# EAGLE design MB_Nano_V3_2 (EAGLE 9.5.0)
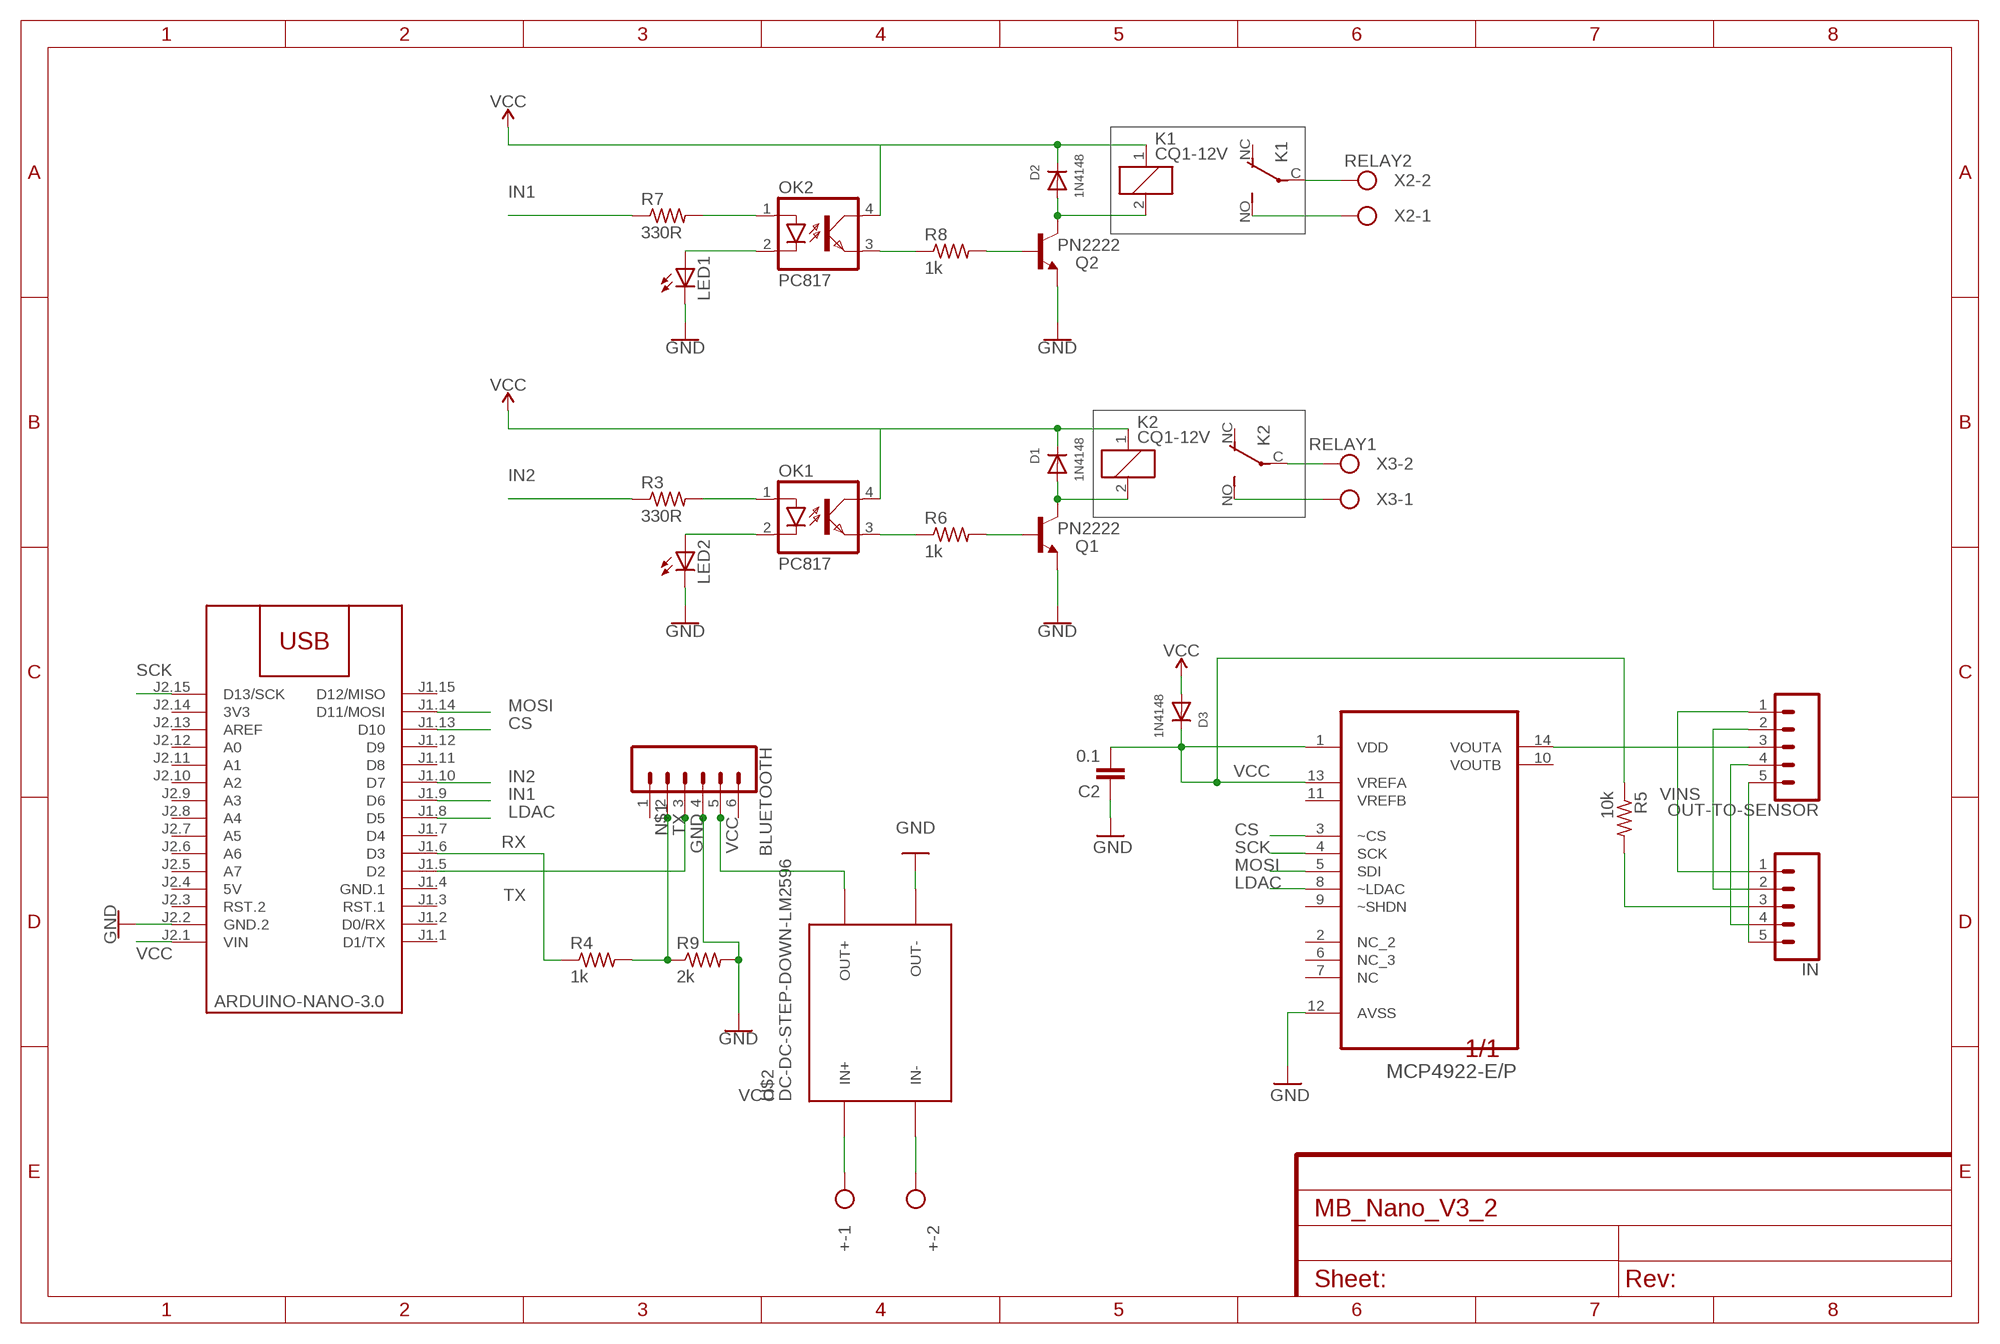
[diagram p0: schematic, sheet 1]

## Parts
+  Vcc  W237-102  [W237-102]
BLUETOOTH  CONN_06LONGPADS  [1X06_LONGPADS]
C2  0.1  CAPPTH1  [CAP-PTH-5MM]
D1  1N4148  DIODEDO-1N4148  [DO-1N4148]
D2  1N4148  DIODEDO-1N4148  [DO-1N4148]
D3  1N4148  DIODEDO-1N4148  [DO-1N4148]
IN  CONN_05PTH_LONGPADS  [1X05_LONGPADS]
K1  CQ1-12V  [CQ1]
K2  CQ1-12V  [CQ1]
LED1  LED3MM  [LED3MM]
LED2  LED3MM  [LED3MM]
M2  ARDUINO-NANO-3.0  [ARDUINO-NANO-3.0]
OK1  PC817  [DIL04]
OK2  PC817  [DIL04]
OUT-TO-SENSOR  CONN_05PTH_LONGPADS  [1X05_LONGPADS]
Q1  PN2222  BC447  [TO92-EBC]
Q2  PN2222  BC447  [TO92-EBC]
R3  330R  R-US_0204/7  [0204/7]
R4  1k  R-US_0204/7  [0204/7]
R5  10k  R-US_0204/7  [0204/7]
R6  1k  R-US_0204/7  [0204/7]
R7  330R  R-US_0204/7  [0204/7]
R8  1k  R-US_0204/7  [0204/7]
R9  2k  R-US_0204/7  [0204/7]
U$2  DC-DC-STEP-DOWN-LM2596  [DC-DC-STEP-DOWN-LM2596]
U$3  MCP4922-E/P  [DIP254P762X533-14]
X2  RELAY2  W237-102  [W237-102]
X3  RELAY1  W237-102  [W237-102]

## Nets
1: IN.5 OUT-TO-SENSOR.5
2: IN.4 OUT-TO-SENSOR.4
4: IN.2 OUT-TO-SENSOR.2
5: IN.1 OUT-TO-SENSOR.1
22: D2.A K1.2 Q2.C
+: +.1 U$2.IN+
-: +.2 U$2.IN-
CS: M2.J1.13(D10) U$3.3(~CS)
GND: BLUETOOTH.4 C2.1 LED1.K(C) LED2.K(C) M2.J2.2(GND.2) Q1.E Q2.E R9.2 U$2.OUT- U$3.12(AVSS)
GND-: D1.A K2.2 Q1.C
IN1: M2.J1.9(D6) R7.1
IN2: M2.J1.10(D7) R3.1
INS: OK1.1(A) R3.2
INSS: OK2.1(A) R7.2
LDAC: M2.J1.8(D5) U$3.8(~LDAC)
LED: LED2.A OK1.2(C)
LEDS: LED1.A OK2.2(C)
MOSI: M2.J1.14(D11/MOSI) U$3.5(SDI)
N$1: BLUETOOTH.2 R4.2 R9.1
N$2: K1.NO(2:S) X2.1
N$3: K1.C(2:P) X2.2
N$4: K2.NO(2:S) X3.1
N$5: K2.C(2:P) X3.2
N$12: Q1.B R6.2
N$20: Q2.B R8.2
N$22: OK2.3(EMIT) R8.1
OTP: OK1.3(EMIT) R6.1
RX: M2.J1.6(D3) R4.1
SCK: M2.J2.15(D13/SCK) U$3.4(SCK)
TX: BLUETOOTH.3 M2.J1.5(D2)
VCC: BLUETOOTH.5 C2.2 D1.C D2.C D3.A D3.C K1.1 K2.1 M2.J2.1(VIN) OK1.4(COL) OK2.4(COL) R5.1 U$2.OUT+ U$3.1(VDD) U$3.13(VREFA)
VINS: IN.3 R5.2
VOUT: OUT-TO-SENSOR.3 U$3.14(VOUTA)
Unconnected: BLUETOOTH.1 BLUETOOTH.6 K1.NC(2:O) K2.NC(2:O) M2.J1.1(D1/TX) M2.J1.2(D0/RX) M2.J1.3(RST.1) M2.J1.7(D4) M2.J1.11(D8) M2.J1.12(D9) M2.J1.15(D12/MISO) M2.J2.3(RST.2) M2.J2.5(A7) M2.J2.6(A6) M2.J2.7(A5) M2.J2.8(A4) M2.J2.9(A3) M2.J2.10(A2) M2.J2.11(A1) M2.J2.12(A0) M2.J2.13(AREF) U$3.2(NC_2) U$3.6(NC_3) U$3.7(NC) U$3.9(~SHDN) U$3.10(VOUTB) U$3.11(VREFB)

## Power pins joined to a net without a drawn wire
3V3: M2.J2.14(3V3)
5V: M2.J2.4(5V)
GND.1: M2.J1.4(GND.1)

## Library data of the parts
+ X2 X3 = con-wago-500:W237-102: WAGO SCREW CLAMP; MPN: 237-102; OC_FARNELL: unknown; OC_NEWARK: 70K9898
BLUETOOTH = SparkFun-Connectors:CONN_06: Multi connection point. Often used as Generic Header-pin footprint for 0.1 inch spaced/style header connections On any of the 0.1 inch spaced packages, you can populate with these: Break Away Headers - Straight (PRT-00116) Break Away Male Headers - Right Angle (PRT-00553) Female Headers (PRT-00115)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
C2 = SparkFun-Passives:CAP: Capacitor
D1-D3 = adafruit:DIODE: Diode
IN OUT-TO-SENSOR = SparkFun-Connectors:CONN_05: Multi connection point. Often used as Generic Header-pin footprint for 0.1 inch spaced/style header connections On any of the 0.1 inch spaced packages, you can populate with these: Break Away Headers - Straight (PRT-00116) Break Away Male Headers - Right Angle (PRT-00553) Female Headers (PRT-00115)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
K1 K2 = relay5vdc:CQ1-12V: AUTOMOTIVE QUIET RELAY NAiS Source: http://www.mew-europe.com/.. en_ds_61208_0000.pdf; OC_FARNELL: unknown; OC_NEWARK: unknown
LED1 LED2 = adafruit:LED: LED
M2 = diy-modules:ARDUINO-NANO-3.0: Arduino Nano 3.0 and compatible devices More details available here: https://www.arduino.cc/en/Main/ArduinoBoardNano Click here to find device on ebay.com
OK1 OK2 = optocoupler:PC817: SHARP OPTO COUPLER; MPN: PC817X4J000F; OC_FARNELL: 9707727; OC_NEWARK: 97K7059
Q1 Q2 = transistor-npn:BC447*: NPN Transistor
R3-R9 = adafruit:R-US_: RESISTOR, American symbol
U$2 = diy-modules:DC-DC-STEP-DOWN-LM2596: DC/DC Step-Down Regulator based on LM2596-ADJ chip LM2596 datasheet available here: http://www.ti.com/lit/ds/symlink/lm2596.pdf Click here to find device on ebay.com
U$3 = Microchip_By_element14_Batch_1:MCP4922-E/P: 12-Bit DAC; MPN: MCP4922-E/P; OC_FARNELL: 1292244; OC_NEWARK: 61K2950; PACKAGE: DIP-14; SUPPLIER: Microchip

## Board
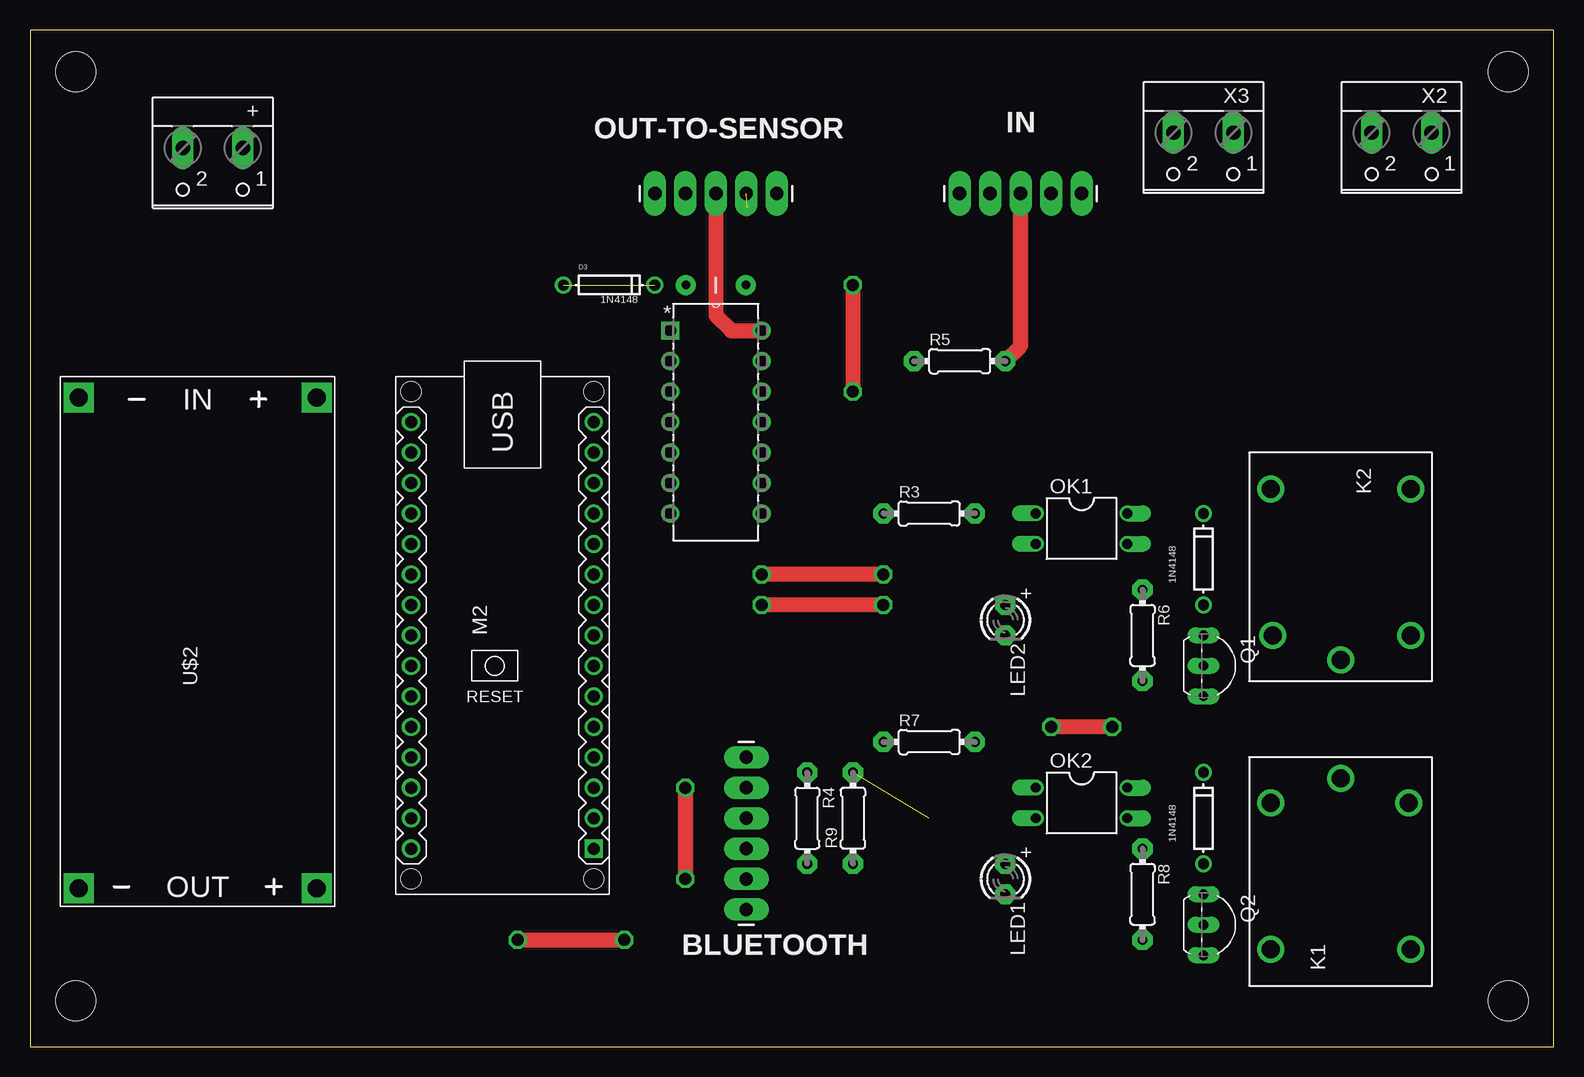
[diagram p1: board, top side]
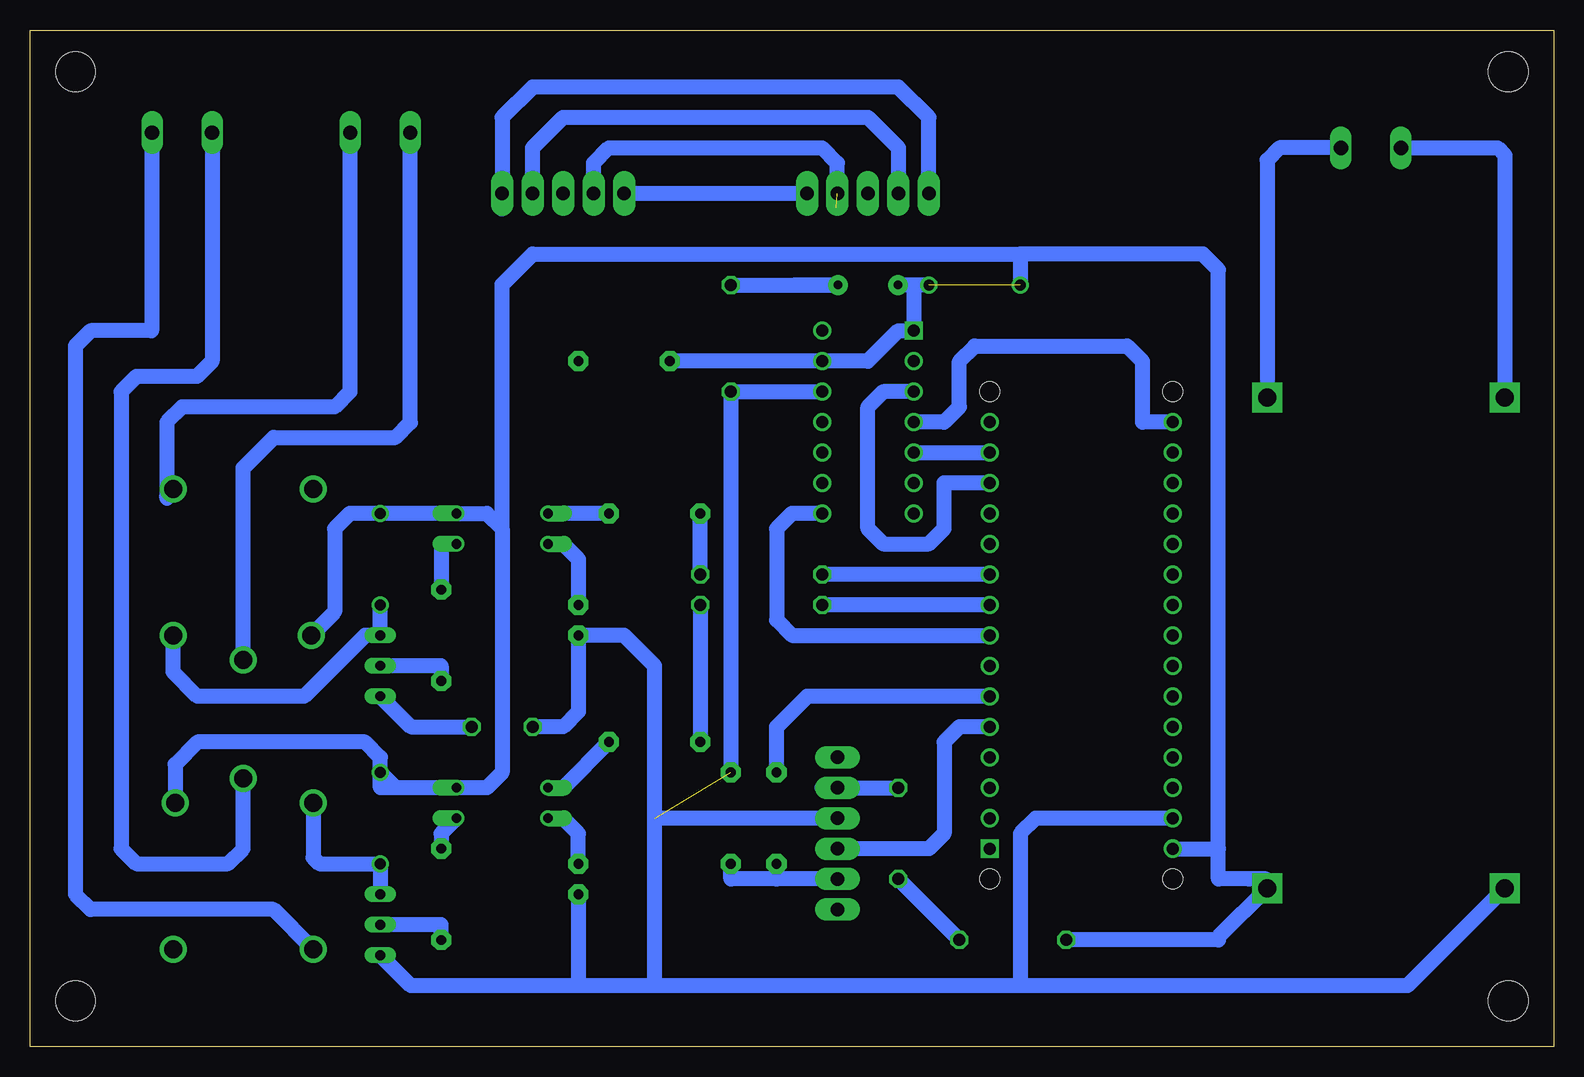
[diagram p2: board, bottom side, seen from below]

Size 126.98 x 84.76 mm. Coordinates in mm from the lower left corner, seen from the top.
Outline: 0,0 126.98,0 126.98,84.76 0,84.76 0,0
Copper layers (1*16): Top 0.035mm / dielectric 1.5mm / Bottom 0.035mm
Design rules "default": minimum track width 6mil, minimum drill 0.35mm, track to track 6mil, track to pad 6mil, pad to pad 6mil, via to via 6mil, smd to smd 6mil, copper to edge 40mil, drill to drill 6mil, minimum pad ring 10mil, minimum via ring 8mil, stop-mask expansion 4mil, vias tented up to drill 0mil, thermal gap 10mil
Holes 3.31 mm at 3.81,3.81 3.81,81.28 123.19,3.81 123.19,81.28

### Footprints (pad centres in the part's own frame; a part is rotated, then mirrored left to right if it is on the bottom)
W237-102 = drill 1.194 long: 1 -2.5,-1.27; 2 2.5,-1.27
1X06_LONGPADS = drill 1.118 pad 1.88 long: 1 0,0; 2 2.54,0; 3 5.08,0; 4 7.62,0; 5 10.16,0; 6 12.7,0
CAP-PTH-5MM = drill 0.7 pad 1.651: 1 -2.5,0; 2 2.5,0
DO-1N4148 = drill 0.9: A -3.81,0; C 3.81,0
1X05_LONGPADS = drill 1.118 pad 1.88 long: 1 0,0; 2 2.54,0; 3 5.08,0; 4 7.62,0; 5 10.16,0
CQ1 = drill 1.5: 1 5.08,-5.66; 2 5.08,5.842; C 7.112,0; NC -7.112,-5.842; NO -7.112,5.842
LED3MM = drill 0.813 pad 1.676 octagon: A -1.27,0; K 1.27,0
ARDUINO-NANO-3.0 = drill 1 square: J1.1 17.78,7.62 | drill 1: J1.2 15.24,7.62; J1.3 12.7,7.62; J1.4 10.16,7.62; J1.5 7.62,7.62; J1.6 5.08,7.62; J1.7 2.54,7.62; J1.8 0,7.62; J1.9 -2.54,7.62; J1.10 -5.08,7.62; J1.11 -7.62,7.62; J1.12 -10.16,7.62; J1.13 -12.7,7.62; J1.14 -15.24,7.62; J1.15 -17.78,7.62; J2.1 17.78,-7.62; J2.2 15.24,-7.62; J2.3 12.7,-7.62; J2.4 10.16,-7.62; J2.5 7.62,-7.62; J2.6 5.08,-7.62; J2.7 2.54,-7.62; J2.8 0,-7.62; J2.9 -2.54,-7.62; J2.10 -5.08,-7.62; J2.11 -7.62,-7.62; J2.12 -10.16,-7.62; J2.13 -12.7,-7.62; J2.14 -15.24,-7.62; J2.15 -17.78,-7.62 | hole 1.651: -20.32,7.62; -20.32,-7.62; 20.32,-7.62; 20.32,7.62
DIL04 = drill 0.813 offset: 1 -1.27,-3.81; 2 1.27,-3.81; 3 1.27,3.81; 4 -1.27,3.81
TO92-EBC = drill 0.813 long: B 0,-1.27; C -2.54,-1.27; E 2.54,-1.27
0204/7 = drill 0.813 pad 1.676 octagon: 1 -3.81,0; 2 3.81,0
DC-DC-STEP-DOWN-LM2596 = drill 1.5 pad 2.5 square: IN+ -22.352,8.636; IN- -22.352,-11.176; OUT+ 18.542,8.636; OUT- 18.542,-11.176
DIP254P762X533-14 = drill 0.991 square: 1 -7.62,15.24 | drill 0.991: 2 -7.62,12.7; 3 -7.62,10.16; 4 -7.62,7.62; 5 -7.62,5.08; 6 -7.62,2.54; 7 -7.62,0; 8 0,0; 9 0,2.54; 10 0,5.08; 11 0,7.62; 12 0,10.16; 13 0,12.7; 14 0,15.24

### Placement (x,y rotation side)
+  15.24,73.66 180 top
BLUETOOTH  59.69,11.43 90 top
C2  57.15,63.5 180 top
D1  97.79,40.64 90 top
D2  97.79,19.05 90 top
D3  48.26,63.5 0 top
IN  87.63,71.12 180 top
K1  109.22,15.24 90 top
K2  109.22,39.37 270 top
LED1  81.28,13.97 270 top
LED2  81.28,35.56 270 top
M2  39.37,34.29 270 top
OK1  87.63,43.18 270 top
OK2  87.63,20.32 270 top
OUT-TO-SENSOR  52.07,71.12 0 top
Q1  99.06,31.75 270 top
Q2  99.06,10.16 270 top
R3  74.93,44.45 0 top
R4  64.77,19.05 270 top
R5  77.47,57.15 0 top
R6  92.71,34.29 270 top
R7  74.93,25.4 0 top
R8  92.71,12.7 270 top
R9  68.58,19.05 90 top
U$2  15.24,31.75 270 top
U$3  60.96,44.45 0 top
X2  114.3,74.93 180 top
X3  97.79,74.93 180 top

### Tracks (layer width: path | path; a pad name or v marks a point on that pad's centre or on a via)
1
  Bottom 1.27: OUT-TO-SENSOR.5 IN.5
2  (1 unrouted)
  Top 0.152: 79.91,71.12 79.91,71.22 IN.4 | 59.79,71.22 OUT-TO-SENSOR.4
  Top 1.27: 59.69,69.85 59.79,69.95
  Bottom 1.27: OUT-TO-SENSOR.4 59.69,73.66 60.96,74.93 78.74,74.93 80.01,73.66 IN.4
4
  Bottom 1.27: IN.2 85.09,74.93 82.55,77.47 57.15,77.47 54.61,74.93 OUT-TO-SENSOR.2
5
  Bottom 1.27: OUT-TO-SENSOR.1 52.07,77.47 54.61,80.01 85.09,80.01 87.63,77.47 IN.1 87.63,69.85
22
  Bottom 1.27: Q2.C D2.A 102.87,15.24 103.38,15.75 K1.2
+
  Bottom 1.27: +.1 22.86,74.93 23.88,73.91 U$2.IN+
-
  Bottom 1.27: +.2 4.68,74.93 4.06,74.32 U$2.IN-
CS
  Bottom 1.27: M2.J1.13 50.8,46.99 50.8,43.18 52.07,41.91 55.88,41.91 57.15,43.18 57.15,53.34 55.88,54.61 U$3.3
GND  (via drill 1)  (1 unrouted)
  Top 1.27: v90.17,26.67 v85.09,26.67 | v68.58,63.5 v68.58,54.61
  Bottom 1.27: Q1.E 95.25,26.67 v90.17,26.67 | U$3.12 v68.58,54.61 R9.2 | M2.J2.2 43.18,19.05 44.45,17.78 44.45,5.08 | v85.09,26.67 82.55,26.67 81.28,27.94 LED2.K 77.47,34.29 74.93,31.75 74.93,19.05 | BLUETOOTH.4 74.93,19.05 | 63.23,63.5 C2.1 v68.58,63.5 | 74.93,5.08 74.93,19.05 | 44.45,5.08 74.93,5.08 | 74.93,5.08 81.28,5.08 | 81.28,5.08 95.25,5.08 Q2.E | LED1.K 81.28,5.08 | U$2.OUT- 12.19,5.08 44.45,5.08
GND-
  Bottom 1.27: D1.A Q1.C 99.06,34.29 104.14,29.21 113.03,29.21 115.06,31.24 K2.2
IN1  (via drill 1)
  Top 1.27: v71.12,36.83 v60.96,36.83
  Bottom 1.27: v71.12,36.83 R7.1 | M2.J1.9 v60.96,36.83
IN2  (via drill 1)
  Top 1.27: v71.12,39.37 v60.96,39.37
  Bottom 1.27: v71.12,39.37 R3.1 | M2.J1.10 v60.96,39.37
INS
  Bottom 1.27: R3.2 OK1.1
INSS
  Bottom 1.27: OK2.1 82.55,21.59 R7.2
LDAC
  Bottom 1.27: M2.J1.8 63.5,34.29 64.77,35.56 64.77,43.18 63.5,44.45 U$3.8
LED
  Bottom 1.27: OK1.2 82.55,41.91 81.28,40.64 LED2.A
LEDS
  Bottom 1.27: LED1.A 81.28,17.78 82.55,19.05 OK2.2
MOSI
  Bottom 1.27: U$3.5 M2.J1.14
N$1
  Bottom 1.27: BLUETOOTH.2 64.77,13.97 | 64.77,13.97 68.58,13.97 R9.1 | R4.2 64.77,13.97
N$2
  Bottom 1.27: K1.NO 106.68,11.43 121.92,11.43 123.19,12.7 123.19,58.42 121.92,59.69 116.84,59.69 116.84,76.16 X2.1 116.8,68.62
N$3
  Bottom 1.27: X2.2 111.8,57.15 113.07,55.88 118.11,55.88 119.38,54.61 119.38,16.51 118.11,15.24 110.49,15.24 109.22,16.51 K1.C
N$4
  Bottom 1.27: 115.57,45.72 115.57,45.97 | 115.57,45.97 K2.NO | 115.57,45.97 115.57,52.07 114.3,53.34 101.6,53.34 100.33,54.61 100.33,76.16 X3.1
N$5
  Bottom 1.27: K2.C 109.22,48.26 106.68,50.8 96.52,50.8 95.29,52.03 X3.2
N$12
  Bottom 1.27: Q1.B 92.71,31.75 R6.2
N$20
  Bottom 1.27: R8.2 92.71,10.16 Q2.B
N$22
  Bottom 1.27: R8.1 92.71,17.78 OK2.3
OTP
  Bottom 1.27: OK1.3 92.71,41.91 R6.1
RX
  Bottom 1.27: M2.J1.6 62.23,29.21 64.77,26.67 R4.1
SCK
  Bottom 1.27: 31.69,52.13 M2.J2.15 34.29,52.07 34.29,57.15 35.56,58.42 48.26,58.42 49.53,57.15 49.53,53.34 50.8,52.07 U$3.4
TX
  Bottom 1.27: BLUETOOTH.3 52.07,16.51 50.8,17.78 50.8,25.4 49.53,26.67 M2.J1.5
VCC  (via drill 0.9, 1)  (1 unrouted)
  Top 1.27: v40.64,8.89 v49.53,8.89 | v54.61,21.59 v54.61,13.97
  Bottom 1.27: 96.52,21.59 OK2.4 88.9,21.59 87.63,22.86 87.63,43.18 | D2.C 96.52,21.59 | M2.J2.1 27.94,16.51 | 25.4,13.97 23.96,13.97 U$2.OUT+ | 87.63,43.18 88.9,44.45 OK1.4 D1.C 100.33,44.45 101.6,43.18 101.6,36.25 K2.1 | 60.96,21.59 BLUETOOTH.5 v54.61,21.59 | v40.64,8.89 27.94,8.89 27.94,9.14 U$2.OUT+ | 96.52,21.59 97.79,21.59 D2.C | D2.C 97.79,24.13 99.06,25.4 113.03,25.4 114.88,23.55 K1.1 | 27.94,16.51 27.94,64.77 29.21,66.04 29.21,66.08 44.45,66.08 | 44.45,66.08 85.09,66.08 87.63,63.54 87.63,43.18 | 44.45,66.08 D3.A | 53.34,63.5 C2.2 | 53.34,63.5 U$3.1 54.61,59.69 57.15,57.15 U$3.13 R5.1 | D3.C 53.34,63.5 | v54.61,13.97 v49.53,8.89 | U$2.OUT+ 24.38,13.97 27.94,13.97 27.94,16.51
  other vias: 52.07,63.5
VINS
  Top 1.27: R5.2 82.55,58.42 IN.3
  Bottom 1.27: R5.2 81.24,57.19
VOUT
  Top 1.27: OUT-TO-SENSOR.3 57.15,60.96 58.42,59.69 U$3.14

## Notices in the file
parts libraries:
diy-modules: Released under the Creative Commons Attribution 4.0 International License: http://creativecommons.org/licenses/by/4.0
SparkFun-PowerSymbols: Licensing: Creative Commons ShareAlike 4.0 International - https://creativecommons.org/licenses/by-sa/4.0
